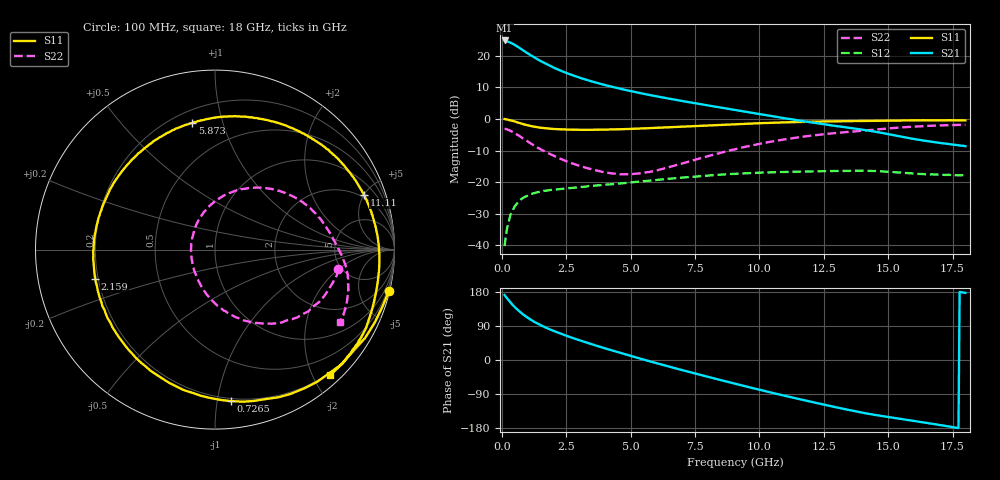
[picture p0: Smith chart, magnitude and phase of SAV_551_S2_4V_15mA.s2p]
! Data provided by Modelithics, Inc.  Tampa, Florida USA, June 2008
!Model SAV-551+
!VAR V_out= 4
!VAR I_out= 15
!VAR V_in= 0.2999
!VAR I_in= 0.8550
!BEGIN ACDATA
# GHZ S MA R 50
! Scattering Parameters
!% F n11x n11y n21x n21y n12x n12y n22x n22y
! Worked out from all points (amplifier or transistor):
!   401 points, 100 MHz to 18 GHz, reference 50 ohm
!   highest |S21| = 24.8 dB at 100 MHz (marker M1)
!   |S21| within 3 dB of that: start of sweep to 796.9 MHz
!   unconditionally stable (mu >= 1): 4.507 GHz to 10.02 GHz; 10.04 GHz to 10.1 GHz; 10.16284 GHz to 10.17481 GHz
!   at 3.054 GHz: K = 0.79, MSG = 17.2 dB, |S12| = -21.5 dB
!   at 9.05 GHz: K = 1.05, MAG = 8.7 dB, |S12| = -17.4 dB
!   at 18 GHz: K = 0.84, MSG = 4.6 dB, |S12| = -17.8 dB
!   lowest NFmin = 0.07 dB at 500 MHz
!   S11 on the Smith chart (normalised r, x): 100 MHz: 0.14, -8.44; 726.5 MHz: 0.18, -1.09; 2.159 GHz: 0.19, -0.12; 5.873 GHz: 0.28, +0.80; 11.11 GHz: 1.80, +5.00; 18 GHz: 0.17, -2.26
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0.1  0.996 -13.5  17.35 171.5  0.00975 81.4  0.6952 -8.9
0.14475  0.9853 -18.8  16.82 167.1  0.01383 80.7  0.6936 -12.0
0.23425  0.9705 -30.4  16.58 159.7  0.02178 72.7  0.6709 -19.5
0.32375  0.9529 -41.8  16.1 152.4  0.03034 67.0  0.6501 -26.6
0.41325  0.931 -52.2  15.41 145.3  0.03543 62.9  0.6232 -33.5
0.5475  0.8961 -66.6  14.33 136.2  0.04414 54.4  0.5788 -42.0
0.7265  0.8486 -84.0  12.84 125.2  0.05306 47.2  0.5197 -52.6
0.995  0.7925 -105.7  10.89 111.6  0.06155 37.4  0.4397 -65.3
1.30825  0.7473 -126.1  9.075 98.8  0.06819 29.2  0.3667 -77.5
1.711  0.7099 -147.3  7.385 85.1  0.07329 21.8  0.2983 -90.2
2.1585  0.6873 -166.1  6.062 72.5  0.07676 16.3  0.245 -102.7
2.56125  0.6769 179.8  5.203 62.3  0.08018 12.4  0.2099 -113.1
3.09825  0.6707 163.4  4.361 49.9  0.08424 7.6  0.1765 -127.3
4.396  0.6825 130.7  3.122 22.6  0.09394 -1.7  0.1362 -166.6
5.87275  0.7164 100.2  2.326 -5.9  0.107 -12.5  0.1488 144.5
6.0965  0.7245 96.1  2.237 -10.1  0.1099 -14.4  0.1573 138.0
7.439  0.7662 73.0  1.782 -34.5  0.1219 -26.0  0.2224 104.5
9.05  0.8211 48.5  1.381 -62.4  0.1356 -41.6  0.3315 74.2
11.1085  0.8836 20.2  1.005 -96.4  0.1454 -64.3  0.4852 42.6
12.04825  0.9031 8.5  0.8759 -110.9  0.1481 -74.8  0.5456 30.2
15.0465  0.9385 -22.8  0.5701 -150.9  0.1457 -105.6  0.7081 -2.9
18  0.945 -47.5  0.3705 177.3  0.1293 -130.7  0.8063 -30.1
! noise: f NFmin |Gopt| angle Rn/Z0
0.5  0.072  0.3861  24.88  0.076
0.7  0.103  0.3941  34.47  0.069
0.9  0.134  0.4018  43.97  0.063
1  0.149  0.4056  48.68  0.06
1.9  0.287  0.4375  89.97  0.042
2.4  0.363  0.4533  112  0.039
3  0.455  0.4705  137.7  0.04
3.9  0.592  0.4927  174.6  0.054
5  0.761  0.514  -143.1  0.091
6  0.914  0.5277  -107.2  0.142
